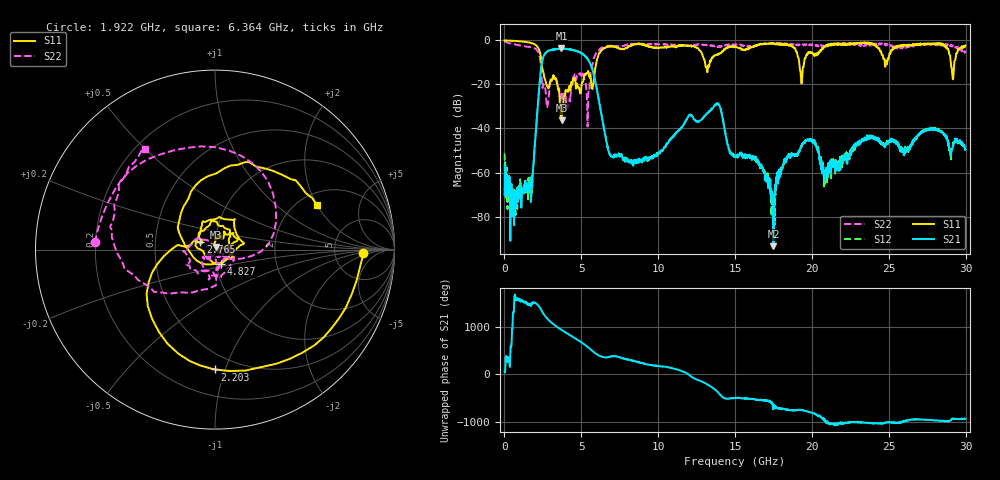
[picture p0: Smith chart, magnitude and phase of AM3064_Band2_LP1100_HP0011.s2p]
# Hz S DB R 50.0
!freq dBS11 angS11 dBS21 angS21 dBS12 angS12 dBS22 angS22
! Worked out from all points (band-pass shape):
!   1600 points, 10 MHz to 29.98 GHz, reference 50 ohm
!   highest |S21| = -3.67 dB at 3.703 GHz (marker M1); lowest = -93.4 dB at 17.5 GHz (marker M2)
!   |S21| within 3 dB of the highest: 2.581 GHz to 5.177 GHz (2.595 GHz wide, 66.9 % of centre)
!   lowest |S11| = -36.3 dB at 3.721 GHz (marker M3), VSWR 1.03, Z = 50.3 + j1.5 ohm
!   |S11| at or under -10 dB: 2.415 GHz to 5.987 GHz (3.572 GHz wide, 85 % of centre); 13.04 GHz to 13.35 GHz (307.3 MHz wide, 2.33 % of centre); 19.17 GHz to 19.49 GHz (325.9 MHz wide, 1.69 % of centre)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
!   |S22| runs from -39.1 to -0.3 dB; largest |S21 - S12| = 0.021
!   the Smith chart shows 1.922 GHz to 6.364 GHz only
!   S11 on the Smith chart (normalised r, x): 1.922 GHz: 10, -1; 2.203 GHz: 0.38, -0.92; 2.765 GHz: 0.85, +0.07; 4.827 GHz: 1.06, -0.17; 6.364 GHz: 2.50, +1.99
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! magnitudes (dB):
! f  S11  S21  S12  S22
! 10 MHz  0.0  -70.0  -51.3  -0.3
! 628.5 MHz  -0.2  -83.9  -78.0  -1.7
! 1.659 GHz  -1.0  -64.5  -64.4  -3.1
! 1.922 GHz  -1.7  -52.7  -52.8  -3.5
! 2.203 GHz  -3.5  -26.5  -26.4  -5.3
! 2.765 GHz  -20.7  -5.1  -5.2  -30.4
! 3.703 GHz  -35.9  -3.7  -3.7  -24.1
! 3.721 GHz  -36.3  -3.8  -3.8  -24.5
! 4.827 GHz  -21.2  -5.2  -5.1  -15.2
! 5.015 GHz  -20.3  -5.9  -5.8  -16.3
! 5.427 GHz  -14.2  -8.7  -8.6  -31.6
! 6.364 GHz  -4.2  -35.7  -35.9  -3.3
! 6.983 GHz  -2.7  -52.8  -53.1  -2.5
! 10 GHz  -3.4  -51.1  -50.9  -1.8
! 13.84 GHz  -6.4  -28.9  -28.6  -2.8
! 15 GHz  -2.7  -52.9  -52.4  -1.8
! 17.5 GHz  -1.5  -93.4  -72.2  -1.1
! 19.33 GHz  -19.6  -47.8  -48.3  -2.2
! 19.99 GHz  -5.4  -45.0  -44.9  -1.8
! 20.91 GHz  -2.3  -60.5  -58.7  -2.5
! 25 GHz  -7.9  -46.1  -45.6  -1.8
! 29.98 GHz  -2.3  -49.6  -48.8  -4.7
